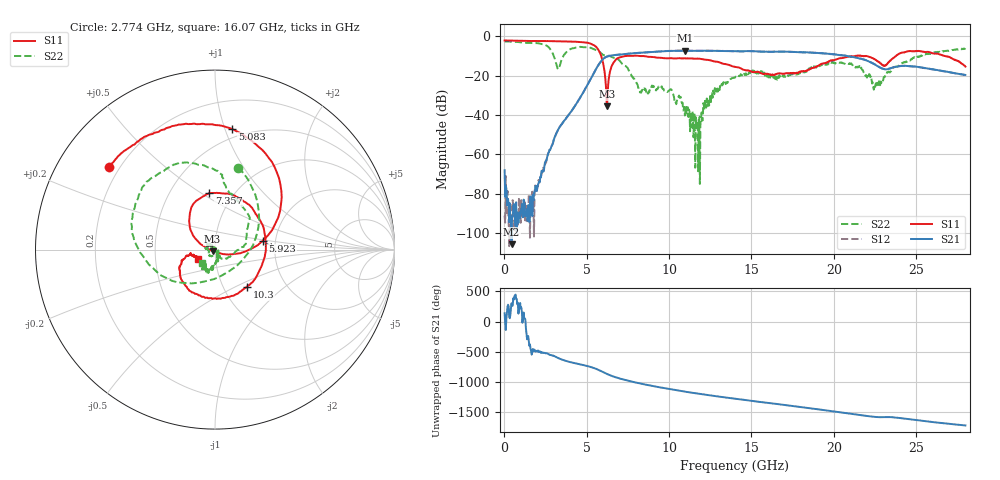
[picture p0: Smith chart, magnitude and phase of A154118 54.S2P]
!  2-Port S-parameters saved by WinCal
! VAR MeasName=S-Parameters (CALIBRATED_DATA) read from VNA (N5230A)
! VAR MeasDate=2015-9-10 14:39:18
! VAR NAME=A154118 54
! VAR FILENAME=A154118 54.S2P
! VAR DATE=2015-9-10 14:39:18
! VAR PHYS_PORTS=1,2
# Hz S DB R 50
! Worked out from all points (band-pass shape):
!   801 points, 10 MHz to 28 GHz, reference 50 ohm
!   highest |S21| = -7.37 dB at 10.96 GHz (marker M1); lowest = -105.9 dB at 429.9 MHz (marker M2)
!   |S21| within 3 dB of the highest: 6.222 GHz to 21 GHz (14.77 GHz wide, 109 % of centre)
!   lowest |S11| = -35.6 dB at 6.238 GHz (marker M3), VSWR 1.03, Z = 48.6 - j0.872 ohm
!   |S11| at or under -10 dB: 5.875 GHz to 7.461 GHz (1.586 GHz wide, 23.8 % of centre); 8.166 GHz to 21.34 GHz (13.17 GHz wide, 89.3 % of centre); 21.95 GHz to 23.79 GHz (1.837 GHz wide, 8.03 % of centre)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
!   |S22| runs from -75.1 to -2.7 dB; largest |S21 - S12| = 0.0078
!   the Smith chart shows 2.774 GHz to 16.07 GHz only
!   S11 on the Smith chart (normalised r, x): 2.774 GHz: 0.16, +0.34; 5.083 GHz: 0.43, +1.06; 5.923 GHz: 1.71, +0.19; 7.357 GHz: 0.77, +0.54; 10.3 GHz: 1.29, -0.58; 16.07 GHz: 0.82, -0.08
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1e7  -2.15 179.7  -68.13 138.7  -91.26 177.7  -2.67 179.8
4.2985e8  -2.22 173.8  -105.85 -56.1  -90.55 77.0  -2.75 169.5
1.864338e9  -2.41 155.4  -78.04 -130.6  -75.94 -103.5  -3.48 132.8
2.774012e9  -2.49 142.1  -57.68 169.2  -57.78 169.5  -6.47 74.2
3.438775e9  -2.58 130.5  -45.11 97.9  -45.11 98.0  -12.76 -125.0
4.698325e9  -3.02 98.2  -29.90 8.8  -29.87 8.9  -5.45 131.8
5.083188e9  -3.37 81.8  -24.11 -17.6  -24.06 -17.5  -5.64 112.9
5.922888e9  -11.33 10.6  -12.21 -104.0  -12.17 -103.9  -8.95 80.1
6.237775e9  -35.64 -147.1  -10.33 -145.7  -10.26 -145.8  -9.84 72.2
7.357375e9  -10.01 95.7  -9.04 114.6  -9.04 114.4  -15.14 10.6
8.26705e9  -10.05 60.7  -8.41 56.6  -8.40 56.4  -28.06 -95.2
9.351662e9  -10.91 5.9  -7.81 -1.0  -7.75 -1.1  -25.62 144.0
1.029632e10  -11.29 -49.5  -7.43 -46.5  -7.38 -46.7  -30.83 137.7
1.096109e10  -11.23 -84.3  -7.37 -75.9  -7.32 -76.5  -40.29 140.3
1.173081e10  -11.32 -118.5  -7.46 -107.6  -7.39 -108.2  -43.25 114.5
1.222064e10  -11.91 -135.7  -7.37 -127.0  -7.33 -127.7  -34.54 -11.6
1.4005e10  -15.57 -166.9  -7.63 167.0  -7.62 166.4  -21.01 -93.9
1.606926e10  -19.28 -152.7  -7.91 95.9  -7.87 95.3  -19.68 -133.9
1.869332e10  -16.12 -115.9  -8.34 5.0  -8.34 4.5  -15.41 -101.7
2.247198e10  -11.50 -162.8  -14.24 -132.3  -14.19 -133.4  -25.68 104.8
2.334666e10  -13.24 -129.4  -16.54 -135.5  -16.55 -137.1  -17.93 -4.8
2.8e10  -15.45 140.3  -19.68 85.6  -19.76 84.6  -6.10 -101.7
